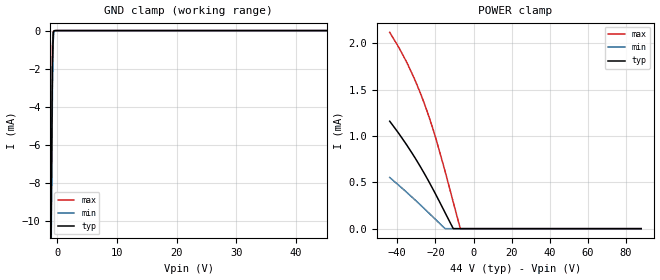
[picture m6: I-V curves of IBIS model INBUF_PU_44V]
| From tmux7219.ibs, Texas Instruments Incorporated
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| Model12
[Model]   INBUF_PU_44V
Model_type   Input
Vinl = 0.8
Vinh = 1.3
|   typ   min   max
C_comp   1.85pF   1.7pF   2.1pF
[Voltage Range]   44   39.6   48.4
[Temperature Range]   27   125   -40
[Power Clamp Reference]   44   39.6   48.4
[GND Clamp Reference]   0   0   0
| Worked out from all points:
|   GND clamp passes 1 mA (typ) near -0.78 V on its own axis
[GND Clamp]
|   Voltage   I(typ)   I(min)   I(max)
-44V      -2.328A    -2.326A    -2.332A
-1.1V     -12.66mA   -14mA      -11.59mA
-968mV    -6.594mA   -8.095mA   -5.409mA
-836mV    -1.77mA    -3.198mA   -813.7uA
-704mV    -86.21uA   -539.1uA   -49.38uA
-572mV    -14.43uA   -27.41uA   -22.26uA
-440mV    -3.065uA   -3.682uA   -4.694uA
88V       0A         0A         0A
[POWER Clamp]
|   Voltage   I(typ)   I(min)   I(max)
-44V      1.159mA    552.6uA    2.118mA
-39.12V   1.024mA    465.8uA    1.952mA
-34.5V    885.3uA    381.3uA    1.771mA
-30.27V   749.2uA    301.8uA    1.581mA
-26.18V   607.8uA    222.7uA    1.37mA
-21.16V   421uA      123.4uA    1.066mA
-19.58V   359.1uA    91.69uA    958.7uA
-15.09V   178.7uA    4.034uA    629.9uA
-10.74V   5.3uA      0A         293.1uA
-7.436V   0A         0A         38.17uA
-6.776V   0A         0A         227.5nA
88V       0A         0A         0A
